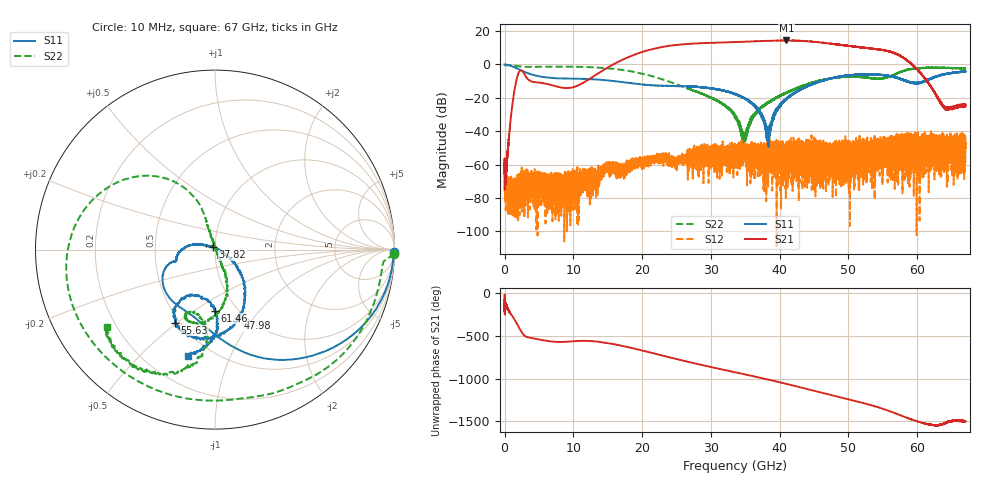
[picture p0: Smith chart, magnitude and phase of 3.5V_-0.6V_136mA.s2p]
! MARKI MICROWAVE INC.
! Date:  10/21/2020
! Model Number:  AMM-7210CH
! Description:  2-port Small Signal S-parameter data for AMM-7210CH
! Frequency Range:  10 MHz to 67 GHz
! Port Configuration:  PORT 1: Input
!  PORT 2: Output
! Bias Condition: Vd = +3.5V, Vg = -0.6V
! AMM-7210CH s2p files are only valid for small signal conditions (below -10 dBm input power)
# Hz S  dB  R 50
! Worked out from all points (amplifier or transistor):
!   20001 points, 10 MHz to 67 GHz, reference 50 ohm
!   highest |S21| = 14.3 dB at 40.97 GHz (marker M1)
!   |S21| within 3 dB of that: 24.31 GHz to 49.55 GHz (25.24 GHz wide, 68.4 % of centre)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
!   unconditionally stable (mu >= 1): start of sweep to 10.00059 MHz; 16.68 MHz to end of sweep
!   at 11.17 GHz: K = 917.92, MAG = -5.6 dB, |S12| = -65.7 dB
!   at 33.51 GHz: K = 73.04, MAG = 13.4 dB, |S12| = -56.8 dB
!   at 67 GHz: K = 382.06, MAG = -19.8 dB, |S12| = -43.4 dB
!   S11 on the Smith chart (normalised r, x): 10 MHz: open; 37.82 GHz: 0.98, +0.02; 47.98 GHz: 0.93, -0.85; 55.63 GHz: 0.47, -0.49; 61.46 GHz: 0.79, -0.61; 67 GHz: 0.38, -0.69
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1e7  -0.01 -0.7  -60.00 -123.5  -61.51 72.0  -0.01 -1.4
2.227369e9  -3.23 -62.6  -3.88 -60.5  -73.51 -42.3  -1.18 -61.7
1.117723e10  -8.63 -132.7  -11.62 161.9  -70.82 152.0  -1.49 -168.6
1.701876e10  -10.54 -159.3  2.49 104.9  -61.49 139.8  -3.29 149.1
1.990938e10  -11.96 -163.7  7.28 51.4  -56.20 117.5  -5.45 129.8
2.234112e10  -12.75 -163.4  9.95 2.5  -56.04 109.2  -8.21 116.8
2.463217e10  -12.96 -164.9  11.45 -43.9  -56.69 90.6  -11.36 109.1
2.764338e10  -13.39 -170.1  12.48 -101.9  -57.75 105.1  -15.95 106.9
3.082205e10  -15.03 178.7  12.96 -159.1  -52.10 34.1  -21.54 106.8
3.3505e10  -17.72 167.5  13.35 153.9  -56.80 107.1  -30.36 98.5
3.782251e10  -35.51 132.1  14.01 77.4  -55.75 30.4  -24.30 -64.7
4.097438e10  -20.53 -30.4  14.30 17.6  -51.52 -45.6  -17.12 -67.4
4.271278e10  -15.72 -38.9  14.19 -17.0  -53.21 170.2  -13.87 -69.1
4.467223e10  -11.96 -49.5  13.68 -56.8  -62.39 -103.4  -10.97 -78.8
4.798489e10  -7.89 -71.1  12.13 -123.1  -62.18 -126.1  -8.00 -95.7
5.139468e10  -6.01 -93.8  10.42 168.7  -53.75 48.7  -7.45 -111.3
5.376613e10  -5.97 -107.8  9.25 117.0  -45.20 -126.6  -8.41 -112.3
5.56251e10  -6.66 -118.8  8.01 68.2  -45.79 -165.4  -7.68 -99.1
5.583612e10  -6.88 -119.8  7.82 62.3  -48.22 -178.7  -7.48 -97.8
5.858271e10  -10.08 -121.0  2.24 -21.8  -48.41 -139.7  -3.34 -103.2
6.145993e10  -9.37 -90.4  -10.28 -92.7  -45.32 -153.8  -2.02 -123.3
6.7e10  -4.46 -105.3  -25.26 -58.5  -43.43 -111.9  -2.50 -144.8
